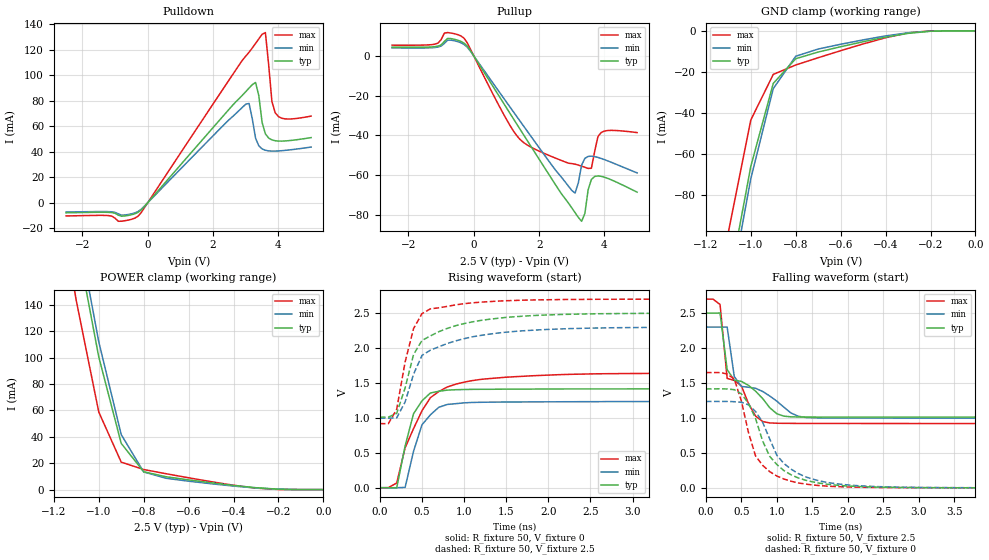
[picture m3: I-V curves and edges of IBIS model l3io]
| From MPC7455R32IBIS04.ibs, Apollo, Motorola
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| *   l3io Model   *
[Model]   l3io
Model_type   I/O
Polarity   Non-Inverting
Vinl = 0.5V
Vinh = 1.7V
Vmeas = 1.25V
Cref = 0
Rref = 50
Vref = 1.25V
|   typ   min   max
C_comp   4.683495e-12   3.353567e-12   5.017392e-12
|   typ   min   max
[Voltage range]   2.5V   2.3V   2.7V
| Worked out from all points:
|   slope of the pulldown table from 0 to 0.375 V, typ, clamps not added: 33.8 ohm
|   slope of the pullup table from 0 to 0.375 V, typ, clamps not added: 38.1 ohm
|   GND clamp passes 1 mA (typ) near -0.28 V on its own axis
|   POWER clamp passes 1 mA (typ) near -0.26 V on its own axis
|   falling waveform, R_fixture 50, V_fixture 2.5: 20-80 % time 535ps typ, 642ps min, 347ps max; typ from 2.5 V to 1.01 V
|   rising waveform, R_fixture 50, V_fixture 0: 20-80 % time 192ps typ, 215ps min, 383ps max; typ from 0.001 V to 1.42 V
|   falling waveform, R_fixture 50, V_fixture 0: 20-80 % time 423ps typ, 467ps min, 319ps max; typ from 1.42 V to 0.001 V
|   rising waveform, R_fixture 50, V_fixture 2.5: 20-80 % time 380ps typ, 438ps min, 208ps max; typ from 1.01 V to 2.5 V
[Pulldown]
|   Voltage   I(typ)   I(min)   I(max)
-2.5V     -7.904mA   -7.296mA   -10.4mA
-300mV    -7.631mA   -6.978mA   -10.67mA
3V        87mA       77.17mA    114.8mA
3.1V      89.77mA    77.75mA    117.9mA
3.3V      94.17mA    50.49mA    124.8mA
3.4V      83.66mA    44.51mA    128.4mA
3.5V      62.75mA    42.13mA    131.9mA
3.6V      53.94mA    41.07mA    133.3mA
3.8V      49.18mA    40.42mA    79.21mA
3.9V      48.54mA    40.43mA    70.49mA
4.2V      48.37mA    40.96mA    65.67mA
5V        50.99mA    43.59mA    67.84mA
[GND_clamp]
-2.5V     -1.152A    -1.159A    -1.15A
-1.1V     -125.1mA   -132mA     -98.3mA
-1V       -66.11mA   -72.14mA   -43.51mA
-900mV    -25.66mA   -28.2mA    -21.26mA
-800mV    -13.6mA    -12.4mA    -16.67mA
-700mV    -10.35mA   -8.884mA   -13.12mA
-600mV    -7.769mA   -6.564mA   -9.691mA
-400mV    -3.094mA   -2.488mA   -3.388mA
-300mV    -1.248mA   -943.2uA   -1.006mA
-200mV    -207.4uA   -146.3uA   0A
0V        0A         0A         0A
[Pullup]
-2.5V     4.444mA    4.048mA    5.415mA
-1.2V     4.639mA    4.223mA    5.89mA
-800mV    8.825mA    7.922mA    11.78mA
-300mV    6.46mA     5.825mA    8.958mA
1.4V      -36.55mA   -32.51mA   -41.84mA
3.1V      -79.03mA   -69.19mA   -54.57mA
3.3V      -83.39mA   -55.04mA   -55.59mA
3.4V      -79.45mA   -51.66mA   -56.16mA
3.6V      -62.29mA   -50.54mA   -56.65mA
3.7V      -60.78mA   -50.77mA   -48.08mA
3.9V      -60.71mA   -51.72mA   -38.59mA
5V        -68.7mA    -59mA      -38.66mA
[POWER_clamp]
-2.5V     1.731A     1.745A     1.708A
-1.2V     290.7mA    303.7mA    243.5mA
-1.1V     190.9mA    203.6mA    143.2mA
-1V       100.7mA    112.1mA    58.86mA
-900mV    35.05mA    41.73mA    20.83mA
-800mV    13.54mA    13.39mA    15.24mA
-700mV    9.739mA    8.569mA    12.03mA
-500mV    5.181mA    4.455mA    6.025mA
-300mV    1.428mA    1.199mA    1.121mA
-200mV    320uA      270.5uA    100.6uA
0V        0A         0A         0A
|   typ   min   max
[Ramp]
dV/dt_r   0.84906/1.63546e-10   0.74103/1.91891e-10   0.98964/3.90035e-10
dV/dt_f   0.89317/5.05156e-10   0.78254/6.21151e-10   1.06865/3.63273e-10
[Falling Waveform]
R_fixture = 50
V_fixture = 2.5
V_fixture_min = 2.3
V_fixture_max = 2.7
| time   V(typ)   V(min)   V(max)
0s        2.5V       2.3V       2.7V
200ps     2.501V     2.3V       2.623V
300ps     1.693V     2.3V       1.566V
400ps     1.54V      1.594V     1.538V
500ps     1.524V     1.451V     1.46V
700ps     1.384V     1.425V     1.028V
900ps     1.147V     1.315V     929.5mV
1.3ns     1.014V     1.026V     922.5mV
1.6ns     1.013V     1.001V     921.9mV
19.7ns    1.011V     995.6mV    918.7mV
[Rising Waveform]
R_fixture = 50
V_fixture = 0
V_fixture_min = 0
V_fixture_max = 0
| time   V(typ)   V(min)   V(max)
0s        824.9uV    802uV      940.9uV
200ps     -1.24mV    897.7uV    68.25mV
300ps     598.6mV    5.107mV    572.1mV
400ps     1.06V      522.4mV    846.9mV
500ps     1.244V     901mV      1.102V
600ps     1.356V     1.044V     1.289V
800ps     1.397V     1.192V     1.442V
1.5ns     1.411V     1.227V     1.582V
3.6ns     1.415V     1.234V     1.638V
19.7ns    1.416V     1.236V     1.65V
[Falling Waveform]
R_fixture = 50
V_fixture = 0
V_fixture_min = 0
V_fixture_max = 0
| time   V(typ)   V(min)   V(max)
0s        1.416V     1.236V     1.65V
400ps     1.405V     1.233V     1.558V
600ps     1.212V     1.189V     794.1mV
700ps     993.7mV    1.093V     458.3mV
800ps     671.4mV    939.3mV    323.1mV
900ps     451.4mV    699.5mV    232.4mV
1.1ns     248.3mV    349.1mV    127.2mV
1.5ns     87.32mV    126.8mV    42mV
3.1ns     3.325mV    5.717mV    3.269mV
19.7ns    855.8uV    763.2uV    1.045mV
[Rising Waveform]
R_fixture = 50
V_fixture = 2.5
V_fixture_min = 2.3
V_fixture_max = 2.7
| time   V(typ)   V(min)   V(max)
0s        1.011V     995.6mV    918.7mV
100ps     1.011V     995.6mV    916.1mV
200ps     1.064V     1V         1.123V
300ps     1.429V     1.228V     1.8V
400ps     1.906V     1.625V     2.277V
500ps     2.107V     1.893V     2.491V
800ps     2.28V      2.064V     2.595V
1.2ns     2.395V     2.18V      2.656V
3.3ns     2.496V     2.295V     2.699V
19.7ns    2.499V     2.299V     2.699V
